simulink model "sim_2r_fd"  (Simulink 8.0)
settings: Solver=ode45  StartTime=0.0  StopTime=1  RelTol=1e-3
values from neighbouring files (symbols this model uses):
  m = 1    [mechanical_system.m]
  s = Lv/norm(Lv)    [pkm1.m]
undefined symbols (not defined in the file or in its folder): deg, kg, N
libraries: mblibv1 x12

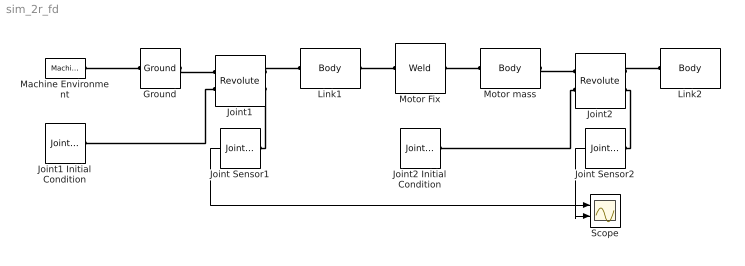
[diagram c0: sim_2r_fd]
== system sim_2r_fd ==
  Ground : mblibv1/Bodies/Ground  UpdateFromCAD=off  LeftPortType=env  RightPortType=workingframe  PhysicalDomain=Mechanical  DialogClass=GroundBlock  CoordPosition=[0 0 0]  CoordPositionUnits=m  StateVectorMgrId=2  MachineId=[3 0]  ShowEnvPort=on
  Joint Sensor1 : mblibv1/Sensors &  Actuators/Joint Sensor  UpdateFromCAD=off  PhysicalDomain=Mechanical  PortType=blob  Muxed=on  Pose=off  Angle=on  AngleUnits=deg  ArcVelocity=off  ArcVelocityUnits=deg/s  ArcAcceleration=off  ArcAccelerationUnits=deg/s^2  CoordPosition=on  CoordPositionUnits=m  Velocity=off  VelocityUnits=m/s  Acceleration=off  AccelerationUnits=m/s^2  Quaternion=on  QuaternionDT=off  QuaternionDDT=off  QuaternionUnits=off  OutputVector=[1]  ActiveIO=on  Width=1  DialogClass=MechanicalSensorBlock  Primitive=R1  Force=off  ForceUnits=N  Torque=off  TorqueUnits=N*m  ReferenceFrame=Absolute (World)  ReactionSensedSide=Base  ReactionReferenceFrame=Absolute (World)  ReactionForce=off  ReactionForceUnits=N  ReactionMoment=off  ReactionMomentUnits=N*m
  Joint Sensor2 : mblibv1/Sensors &  Actuators/Joint Sensor  UpdateFromCAD=off  PhysicalDomain=Mechanical  PortType=blob  Muxed=on  Pose=off  Angle=on  AngleUnits=deg  ArcVelocity=off  ArcVelocityUnits=deg/s  ArcAcceleration=off  ArcAccelerationUnits=deg/s^2  CoordPosition=on  CoordPositionUnits=m  Velocity=off  VelocityUnits=m/s  Acceleration=off  AccelerationUnits=m/s^2  Quaternion=on  QuaternionDT=off  QuaternionDDT=off  QuaternionUnits=off  OutputVector=[1]  ActiveIO=on  Width=1  DialogClass=MechanicalSensorBlock  Primitive=R1  Force=off  ForceUnits=N  Torque=off  TorqueUnits=N-m  ReferenceFrame=Absolute (World)  ReactionSensedSide=Base  ReactionReferenceFrame=Absolute (World)  ReactionForce=off  ReactionForceUnits=N  ReactionMoment=off  ReactionMomentUnits=N-m
  Joint1 : mblibv1/Joints/Revolute  LConnTagsString=__newl0|SA1  RConnTagsString=__newr0|SA1  UpdateFromCAD=off  NumSAPorts=2  CutJoint=off  MarkAsCut=off  Primitives=prismatic  PrimitiveProps=R1$World$[0 0 1]$revolute  DialogClass=JointBlock  R1Axis=[0 0 1]
  Joint1 Initial Condition : mblibv1/Sensors &  Actuators/Joint Initial Condition  UpdateFromCAD=off  LeftPortType=blob  RightPortType=blob  PhysicalDomain=mechanical  DialogClass=InitialConditionBlock  InitialConditions=P1$false$0$m$deg$0$m/s$deg/s#P2$false$0$m$deg$0$m/s$deg/s#P3$false$0$m$deg$0$m/s$deg/s#R1$true$-60$m$deg$0$m/s$deg/s#R2$false$0$m$deg$0$m/s$deg/s#R3$false$0$m$deg$0$m/s$deg/s#S$false$0$m$deg$0$m/s$deg/s  P1PIC=0  P1VIC=0  P2PIC=0  P2VIC=0  P3PIC=0  P3VIC=0  R1PIC=-60  R1VIC=0  R2PIC=0  R2VIC=0  R3PIC=0  R3VIC=0  SPIC=0  SVIC=0
  Joint2 : mblibv1/Joints/Revolute  LConnTagsString=__newl0|SA1  RConnTagsString=__newr0|SA1  UpdateFromCAD=off  NumSAPorts=2  CutJoint=off  MarkAsCut=off  Primitives=prismatic  PrimitiveProps=R1$World$[0 0 1]$revolute  DialogClass=JointBlock  R1Axis=[0 0 1]
  Joint2 Initial Condition : mblibv1/Sensors &  Actuators/Joint Initial Condition  UpdateFromCAD=off  LeftPortType=blob  RightPortType=blob  PhysicalDomain=mechanical  DialogClass=InitialConditionBlock  InitialConditions=P1$false$0$m$deg$0$m/s$deg/s#P2$false$0$m$deg$0$m/s$deg/s#P3$false$0$m$deg$0$m/s$deg/s#R1$false$0$m$deg$0$m/s$deg/s#R2$false$0$m$deg$0$m/s$deg/s#R3$false$0$m$deg$0$m/s$deg/s#S$false$0$m$deg$0$m/s$deg/s  P1PIC=0  P1VIC=0  P2PIC=0  P2VIC=0  P3PIC=0  P3VIC=0  R1PIC=0  R1VIC=0  R2PIC=0  R2VIC=0  R3PIC=0  R3VIC=0  SPIC=0  SVIC=0
  Link1 : mblibv1/Bodies/Body  LConnTagsString=CS1  RConnTagsString=CS2  UpdateFromCAD=off  DialogClass=MechanicalBodyBlock  Mass=0.071  MassUnits=kg  InertiaUnits=kg*m^2  Inertia=[0 0 0; 0 0 0; 0 0 0.000089395]  Shape=Cylinder  ShapeDims=[1 1]  ShapeUnits=m  ShapeUse=false  Density=1  DensityUnits=kg/m^3  DensityUse=false  GraphicsMode=MACHINE_DEFAULT  BodyColorSelMode=MACHINE_DEFAULT  BodyColor=[1 0 0]  AttachedToCS=CG  CG=Left$CG$[0.0373 0 0]$CS1$CS1$m$[0 0 0]$Euler X-Y-Z$deg$WORLD$false$none  WorkingFrames=Left$CS1$[0 0 0]$World$World$m$[0 0 0]$Euler X-Y-Z$deg$WORLD$true$none#Right$CS2$[0.1 0 0]$World$World$m$[0 0 0]$Euler X-Y-Z$deg$WORLD$true$none  CGPos=[0.0373 0 0]  CGRot=[0 0 0]  CS0Pos=[]  CS0Rot=[]  CS1Pos=[0 0 0]  CS1Rot=[0 0 0]  CS2Pos=[0.1 0 0]  CS2Rot=[0 0 0]  CS3Pos=[]  CS3Rot=[]  CS4Pos=[]  CS4Rot=[]  CS5Pos=[]  CS5Rot=[]  CS6Pos=[]  CS6Rot=[]  CS7Pos=[]  CS7Rot=[]  CS8Pos=[]  CS8Rot=[]  CS9Pos=[]  CS9Rot=[]  CS10Pos=[]  CS10Rot=[]  CS11Pos=[]  CS11Rot=[]  CS12Pos=[]  CS12Rot=[]  CS13Pos=[]  CS13Rot=[]  CS14Pos=[]  CS14Rot=[]  CS15Pos=[]  CS15Rot=[]  CS16Pos=[]  CS16Rot=[]  CS17Pos=[]  CS17Rot=[]  CS18Pos=[]  CS18Rot=[]  CS19Pos=[]  CS19Rot=[]  CS20Pos=[]  CS20Rot=[]
  Link2 : mblibv1/Bodies/Body  LConnTagsString=CS1  UpdateFromCAD=off  DialogClass=MechanicalBodyBlock  Mass=0.1  MassUnits=kg  InertiaUnits=kg*m^2  Inertia=[0 0 0; 0 0 0; 0 0 0.000109864]  Shape=Cylinder  ShapeDims=[1 1]  ShapeUnits=m  ShapeUse=false  Density=1  DensityUnits=kg/m^3  DensityUse=false  GraphicsMode=MACHINE_DEFAULT  BodyColorSelMode=MACHINE_DEFAULT  BodyColor=[1 0 0]  AttachedToCS=CG  CG=Left$CG$[0.04168 0 0]$CS1$CS1$m$[0 0 0]$Euler X-Y-Z$deg$WORLD$false$none  WorkingFrames=Left$CS1$[0.1 0 0]$World$World$m$[0 0 0]$Euler X-Y-Z$deg$WORLD$true$none#Right$CS2$[0.2 0 0]$World$World$m$[0 0 0]$Euler X-Y-Z$deg$WORLD$false$none  CGPos=[0.04168 0 0]  CGRot=[0 0 0]  CS0Pos=[]  CS0Rot=[]  CS1Pos=[0.1 0 0]  CS1Rot=[0 0 0]  CS2Pos=[0.2 0 0]  CS2Rot=[0 0 0]  CS3Pos=[]  CS3Rot=[]  CS4Pos=[]  CS4Rot=[]  CS5Pos=[]  CS5Rot=[]  CS6Pos=[]  CS6Rot=[]  CS7Pos=[]  CS7Rot=[]  CS8Pos=[]  CS8Rot=[]  CS9Pos=[]  CS9Rot=[]  CS10Pos=[]  CS10Rot=[]  CS11Pos=[]  CS11Rot=[]  CS12Pos=[]  CS12Rot=[]  CS13Pos=[]  CS13Rot=[]  CS14Pos=[]  CS14Rot=[]  CS15Pos=[]  CS15Rot=[]  CS16Pos=[]  CS16Rot=[]  CS17Pos=[]  CS17Rot=[]  CS18Pos=[]  CS18Rot=[]  CS19Pos=[]  CS19Rot=[]  CS20Pos=[]  CS20Rot=[]
  Machine Environment : mblibv1/Bodies/Machine Environment  PortType=env  PhysicalDomain=Mechanical  DialogTemplateClass=MECH.MachineEnvironment  SyncWhenCopied=off  Gravity=[0 -9.81 0]  GravityUnits=m/s^2  GravityAsSignal=off  Dimensionality=Auto-detect  AnalysisType=Forward dynamics  LinearAssemblyTolerance=1e-3  LinearAssemblyToleranceUnits=m  AngularAssemblyTolerance=1e-3  AngularAssemblyToleranceUnits=rad  ConstraintSolverType=Stabilizing  ConstraintRelTolerance=1e-4  ConstraintAbsTolerance=1e-4  UseRobustSingularityHandling=off  RedundancyAnalysisToleranceType=Automatically select tolerance  RedundancyAnalysisTolerance=1e-14  StatePerturbationType=Fixed  PerturbationSize=1e-5  VisualizeMachine=on  BodyVisualizationType=Use model default body geometries  BodyColorSelMode=Use model default  DefaultBodyColor=[1 0 0]
  Motor Fix : mblibv1/Joints/Weld  LConnTagsString=__newl0  RConnTagsString=__newr0  UpdateFromCAD=off  NumSAPorts=0  CutJoint=off  MarkAsCut=off  Primitives=weld  PrimitiveProps=W$WORLD$[0 0 0]$weld  DialogClass=JointBlock  WAxis=[0 0 0]
  Motor mass : mblibv1/Bodies/Body  LConnTagsString=CS1  RConnTagsString=CS2  UpdateFromCAD=off  DialogClass=MechanicalBodyBlock  Mass=0.292  MassUnits=kg  InertiaUnits=kg*m^2  Inertia=[0 0 0; 0 0 0; 0 0 0]  Shape=Cylinder  ShapeDims=[1 1]  ShapeUnits=m  ShapeUse=false  Density=1  DensityUnits=kg/m^3  DensityUse=false  GraphicsMode=MACHINE_DEFAULT  BodyColorSelMode=MACHINE_DEFAULT  BodyColor=[1 0 0]  AttachedToCS=CG  CG=Left$CG$[0.1 0 0]$WORLD$WORLD$m$[0 0 0]$Euler X-Y-Z$deg$WORLD$false$none  WorkingFrames=Left$CS1$[0.1 0 0]$World$World$m$[0 0 0]$Euler X-Y-Z$deg$WORLD$true$none#Right$CS2$[0.1 0 0]$World$World$m$[0 0 0]$Euler X-Y-Z$deg$WORLD$true$none  CGPos=[0.1 0 0]  CGRot=[0 0 0]  CS0Pos=[]  CS0Rot=[]  CS1Pos=[0.1 0 0]  CS1Rot=[0 0 0]  CS2Pos=[0.1 0 0]  CS2Rot=[0 0 0]  CS3Pos=[]  CS3Rot=[]  CS4Pos=[]  CS4Rot=[]  CS5Pos=[]  CS5Rot=[]  CS6Pos=[]  CS6Rot=[]  CS7Pos=[]  CS7Rot=[]  CS8Pos=[]  CS8Rot=[]  CS9Pos=[]  CS9Rot=[]  CS10Pos=[]  CS10Rot=[]  CS11Pos=[]  CS11Rot=[]  CS12Pos=[]  CS12Rot=[]  CS13Pos=[]  CS13Rot=[]  CS14Pos=[]  CS14Rot=[]  CS15Pos=[]  CS15Rot=[]  CS16Pos=[]  CS16Rot=[]  CS17Pos=[]  CS17Rot=[]  CS18Pos=[]  CS18Rot=[]  CS19Pos=[]  CS19Rot=[]  CS20Pos=[]  CS20Rot=[]
  Scope : Scope  NumInputPorts=2
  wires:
  Joint Sensor1/1 -> Scope/1
  Joint Sensor2/1 -> Scope/2
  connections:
  Machine Environment/RConn1 -- Ground/LConn1
  Joint1/RConn1 -- Link1/LConn1
  Ground/RConn1 -- Joint1/LConn1
  Link1/RConn1 -- Motor Fix/LConn1
  Motor Fix/RConn1 -- Motor mass/LConn1
  Motor mass/RConn1 -- Joint2/LConn1
  Joint2/RConn1 -- Link2/LConn1
  Joint1/LConn2 -- Joint1 Initial Condition/RConn1
  Joint2/LConn2 -- Joint2 Initial Condition/RConn1
  Joint1/RConn2 -- Joint Sensor1/LConn1
  Joint2/RConn2 -- Joint Sensor2/LConn1
